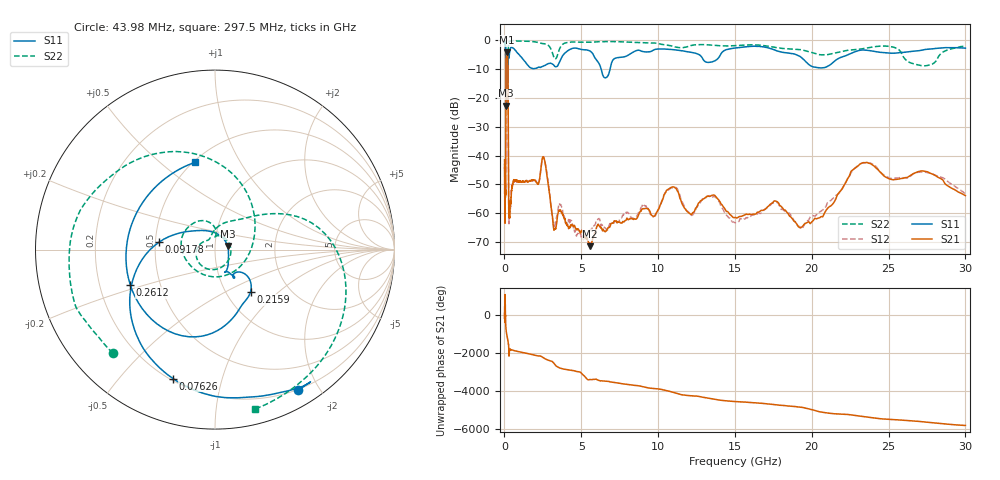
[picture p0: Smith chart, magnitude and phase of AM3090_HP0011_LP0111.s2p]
! Date/Time: Thu, Feb 28, 2019 1:56 PM
! Network Analyzer: Agilent Technologies E8364B Rev: A.07.50.67
! Sweep from 0.010 to 30.000 GHz, 1601 Points, Sweep Type: LOG
! Power Supply: 5.022 V, 0.002 A
# Hz S DB R 50
!freq MagS11 AngS11 MagS21 AngS21 MagS12 AngS12 MagS22 AngS22
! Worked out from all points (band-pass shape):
!   1601 points, 10 MHz to 30 GHz, reference 50 ohm
!   highest |S21| = -4.26 dB at 151.4 MHz (marker M1); lowest = -71.4 dB at 5.584 GHz (marker M2)
!   |S21| within 3 dB of the highest: 102.8 MHz to 217 MHz (114.2 MHz wide, 71.4 % of centre)
!   lowest |S11| = -22.8 dB at 100.4 MHz (marker M3), VSWR 1.16, Z = 57.5 + j2.26 ohm
!   |S11| at or under -10 dB: 91.76 MHz to 217.6 MHz (125.8 MHz wide, 81.4 % of centre); 6.288 GHz to 6.877 GHz (588.6 MHz wide, 8.94 % of centre)
!   |S22| runs from -23.7 to -0.2 dB; largest |S21 - S12| = 0.011
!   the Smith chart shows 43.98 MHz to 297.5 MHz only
!   S11 on the Smith chart (normalised r, x): 43.98 MHz: 0.19, -1.74; 76.26 MHz: 0.21, -0.71; 91.78 MHz: 0.52, +0.05; 215.9 MHz: 1.29, -0.68; 261.2 MHz: 0.33, -0.18; 297.5 MHz: 0.51, +0.66
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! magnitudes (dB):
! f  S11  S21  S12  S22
! 10 MHz  -0.2  -41.5  -43.1  -0.6
! 38.04 MHz  -0.5  -59.9  -59.1  -1.5
! 43.98 MHz  -0.8  -58.9  -57.1  -1.8
! 76.26 MHz  -2.4  -50.1  -47.8  -4.4
! 91.78 MHz  -10.0  -16.1  -16.1  -16.2
! 100.4 MHz  -22.8  -8.1  -8.1  -14.1
! 144.7 MHz  -15.4  -4.3  -4.3  -21.4
! 151.4 MHz  -15.2  -4.3  -4.2  -20.9
! 215.9 MHz  -10.2  -7.1  -7.1  -16.9
! 235.1 MHz  -7.8  -15.2  -15.2  -8.9
! 261.2 MHz  -5.8  -46.5  -46.9  -1.8
! 297.5 MHz  -6.0  -60.7  -63.6  -0.8
! 550.5 MHz  -2.8  -49.6  -49.9  -0.3
! 2.084 GHz  -9.8  -49.3  -49.3  -0.7
! 2.558 GHz  -9.0  -40.6  -40.7  -1.3
! 3.253 GHz  -9.0  -65.7  -64.5  -6.4
! 5.584 GHz  -3.9  -71.4  -65.7  -0.8
! 7.926 GHz  -5.6  -62.3  -59.6  -0.7
! 10.86 GHz  -3.3  -51.0  -51.2  -2.1
! 19.7 GHz  -8.0  -63.2  -62.6  -3.9
! 23.48 GHz  -3.5  -42.5  -42.6  -2.9
! 30 GHz  -2.8  -53.9  -53.3  -2.2
